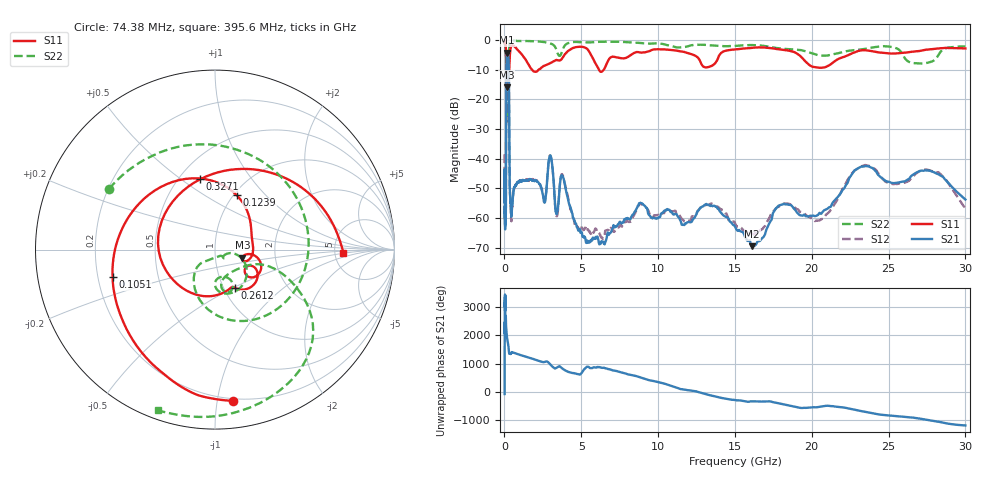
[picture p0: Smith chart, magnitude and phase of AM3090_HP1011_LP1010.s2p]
! Date/Time: Thu, Feb 28, 2019 2:05 PM
! Network Analyzer: Agilent Technologies E8364B Rev: A.07.50.67
! Sweep from 0.010 to 30.000 GHz, 1601 Points, Sweep Type: LOG
! Power Supply: 5.023 V, 0.002 A
# Hz S DB R 50
!freq MagS11 AngS11 MagS21 AngS21 MagS12 AngS12 MagS22 AngS22
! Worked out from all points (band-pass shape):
!   1601 points, 10 MHz to 30 GHz, reference 50 ohm
!   highest |S21| = -4.27 dB at 176.8 MHz (marker M1); lowest = -69.4 dB at 16.13 GHz (marker M2)
!   |S21| within 3 dB of the highest: 131.3 MHz to 274.6 MHz (143.3 MHz wide, 70.6 % of centre)
!   lowest |S11| = -16.0 dB at 159.1 MHz (marker M3), VSWR 1.38, Z = 67.7 - j6.15 ohm
!   |S11| at or under -10 dB: 124.4 MHz to 308.8 MHz (184.3 MHz wide, 85.1 % of centre); 1.792 GHz to 2.229 GHz (437.2 MHz wide, 21.7 % of centre); 6.146 GHz to 6.465 GHz (319.3 MHz wide, 5.06 % of centre)
!   |S22| runs from -27.6 to -0.2 dB; largest |S21 - S12| = 0.015
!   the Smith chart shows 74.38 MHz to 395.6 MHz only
!   S11 on the Smith chart (normalised r, x): 74.38 MHz: 0.18, -1.11; 105.1 MHz: 0.26, -0.12; 123.9 MHz: 1.03, +0.70; 261.2 MHz: 1.13, -0.51; 327.1 MHz: 0.63, +0.59; 395.6 MHz: 5.99, -0.41
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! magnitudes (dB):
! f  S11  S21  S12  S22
! 10 MHz  -0.2  -45.6  -38.5  -0.7
! 38.04 MHz  -0.4  -60.0  -59.5  -1.5
! 74.38 MHz  -1.4  -53.9  -56.9  -3.3
! 91.78 MHz  -2.8  -57.1  -56.2  -4.9
! 105.1 MHz  -4.6  -38.6  -38.9  -5.6
! 123.9 MHz  -9.7  -11.6  -11.6  -13.1
! 144.7 MHz  -13.8  -5.2  -5.1  -23.6
! 159.1 MHz  -16.0  -4.5  -4.4  -21.0
! 176.8 MHz  -12.3  -4.3  -4.2  -13.1
! 261.2 MHz  -12.4  -5.9  -5.8  -14.3
! 327.1 MHz  -8.0  -45.3  -44.6  -1.3
! 395.6 MHz  -2.9  -54.7  -55.5  -0.4
! 550.5 MHz  -1.9  -52.8  -52.6  -0.3
! 2.084 GHz  -10.7  -47.5  -47.2  -0.5
! 2.987 GHz  -7.7  -38.9  -38.9  -1.2
! 3.368 GHz  -6.7  -58.4  -59.2  -3.1
! 3.779 GHz  -6.0  -45.7  -45.4  -3.5
! 5.311 GHz  -2.7  -68.3  -62.6  -0.8
! 7.926 GHz  -6.0  -60.0  -61.0  -0.7
! 16.13 GHz  -2.6  -69.4  -65.2  -1.7
! 23.36 GHz  -3.4  -42.6  -42.3  -3.1
! 30 GHz  -2.9  -53.7  -56.7  -2.2
